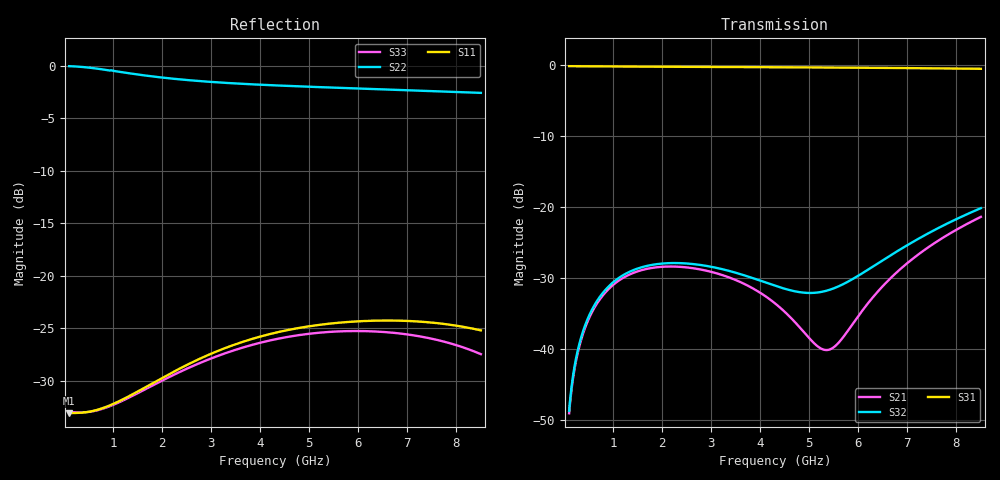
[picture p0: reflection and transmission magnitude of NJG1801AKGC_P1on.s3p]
! Port1:P1, Port2:P2, Port3:PC, VCTL1=0V, VCTL2=3V
# hz S ma R 50
! 3 Port Network Data from SP1.SP block
! freq  magS11  angS11  magS12  angS12  magS13  angS13
!  magS21  angS21
!  magS22  angS22  magS23  angS23
!  magS31  angS31  magS32  angS32
!  magS33  angS33
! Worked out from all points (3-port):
!   841 points, 100 MHz to 8.5 GHz, reference 50 ohm
!   strongest paths, dB at 100 MHz, 2.2 GHz, 4.3 GHz, 6.4 GHz, 8.5 GHz:
!     S31: -0.2, -0.3, -0.4, -0.5, -0.6
!     S32: -48.8, -28.0, -31.1, -28.0, -20.2
!     S21: -49.1, -28.4, -33.6, -32.0, -21.5
!   lowest |S11| = -33.1 dB at 100 MHz (marker M1), VSWR 1.05, Z = 52.3 - j0.147 ohm
!   |S11| at or under -10 dB: start of sweep to end of sweep
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1e8  0.02217 -3.6  0.003502 74.3  0.9738 -1.1
     0.0035 74.4  0.9945 -7.4  0.003643 74.6
     0.9738 -1.1  0.003645 74.5  0.02231 -3.0
2.7e8  0.02225 -11.1  0.009144 73.9  0.9729 -3.0
       0.009142 73.9  0.99 -19.8  0.009499 74.6
       0.9729 -3.0  0.009501 74.6  0.02241 -11.4
5.2e8  0.02258 -21.7  0.01676 65.5  0.9714 -5.7
       0.01675 65.6  0.9777 -37.6  0.01742 66.6
       0.9714 -5.7  0.01742 66.6  0.02254 -23.1
9.4e8  0.02423 -38.3  0.02693 50.5  0.9692 -10.2
       0.02693 50.5  0.9484 -65.3  0.02806 52.2
       0.9692 -10.2  0.02806 52.2  0.02401 -40.9
1.37e9  0.02711 -52.5  0.03367 36.9  0.9674 -14.7
        0.03366 36.9  0.9167 -89.5  0.03518 39.6
        0.9674 -14.7  0.03519 39.6  0.02668 -56.5
2.63e9  0.03894 -80.6  0.0368 7.7  0.9634 -28.1
        0.03679 7.7  0.8496 -142.2  0.03935 14.5
        0.9634 -28.1  0.03936 14.5  0.03727 -89.9
4.3e9  0.05354 -103.7  0.02082 -8.9  0.9574 -46.1
       0.02082 -8.9  0.8057 171.5  0.0277 11.1
       0.9574 -46.1  0.02771 11.1  0.04985 -121.5
5.43e9  0.05926 -115.4  0.009897 45.5  0.9526 -58.5
        0.009894 45.5  0.7871 146.4  0.02603 40.4
        0.9526 -58.5  0.02604 40.4  0.05412 -140.3
6.87e9  0.06114 -127.0  0.03662 90.3  0.945 -74.6
        0.03662 90.3  0.7661 117.1  0.05028 61.1
        0.9451 -74.6  0.05029 61.1  0.05308 -164.7
8.5e9  0.055 -135.3  0.0846 76.4  0.9331 -93.6
       0.0846 76.4  0.7422 85.0  0.09743 51.5
       0.9331 -93.6  0.09744 51.5  0.04238 161.0
